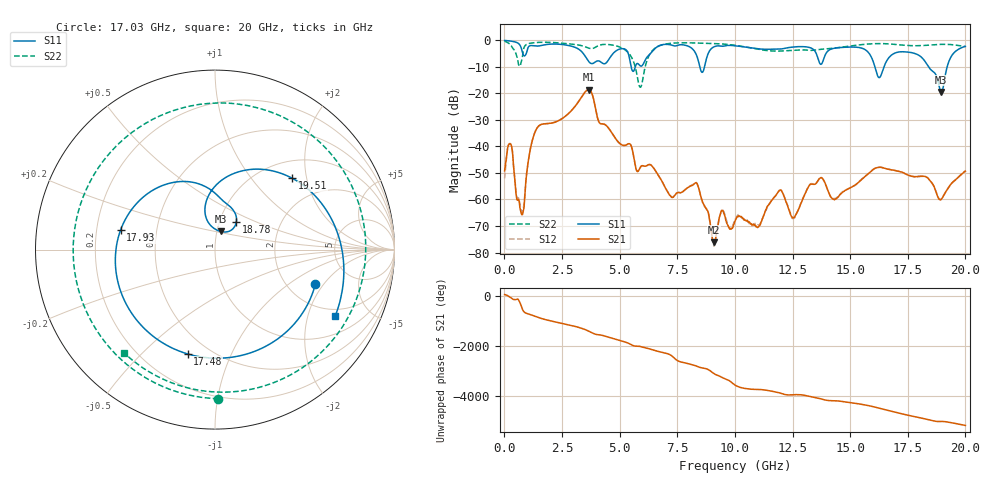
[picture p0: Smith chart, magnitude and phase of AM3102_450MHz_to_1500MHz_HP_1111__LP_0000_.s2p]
!Agilent Technologies,E8364B,MY43040894,A.07.50.67
!Agilent E8364B: A.07.50.67
!Date: Thursday, January 11, 2018 06:48:17
!Correction: S11(Full 2 Port(1,2))
!S21(Full 2 Port(1,2))
!S12(Full 2 Port(1,2))
!S22(Full 2 Port(1,2))
!S2P File: Measurements: S11, S21, S12, S22:
# Hz S  dB  R 50
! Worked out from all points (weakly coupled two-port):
!   1601 points, 10 MHz to 20 GHz, reference 50 ohm
!   highest |S21| = -18.60 dB at 3.658 GHz (marker M1); lowest = -76.1 dB at 9.08 GHz (marker M2)
!   lowest |S11| = -19.5 dB at 18.95 GHz (marker M3), VSWR 1.24, Z = 52.1 + j10.6 ohm
!   |S11| at or under -10 dB: 8.477 GHz to 8.682 GHz (204.6 MHz wide, 2.38 % of centre); 16.07 GHz to 16.47 GHz (396 MHz wide, 2.43 % of centre); 18.4 GHz to 19.21 GHz (809.2 MHz wide, 4.3 % of centre)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
!   |S22| runs from -17.7 to -0.4 dB; largest |S21 - S12| = 0.0015
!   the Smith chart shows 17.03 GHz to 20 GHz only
!   S11 on the Smith chart (normalised r, x): 17.03 GHz: 2.83, -1.65; 17.48 GHz: 0.38, -0.70; 17.93 GHz: 0.30, +0.09; 18.78 GHz: 1.20, +0.38; 19.51 GHz: 1.36, +1.65; 20 GHz: 1.68, -3.01
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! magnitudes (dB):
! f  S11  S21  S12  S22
! 10 MHz  -0.1  -49.3  -52.0  -0.4
! 259.9 MHz  -0.3  -39.1  -39.0  -1.6
! 772.1 MHz  -4.1  -65.8  -64.8  -6.6
! 1.384 GHz  -2.2  -33.6  -33.6  -0.8
! 3.346 GHz  -4.2  -21.4  -21.4  -2.0
! 3.658 GHz  -8.0  -18.6  -18.6  -2.9
! 5.895 GHz  -9.6  -47.9  -47.9  -17.7
! 6.682 GHz  -2.2  -50.9  -51.0  -2.2
! 8.343 GHz  -5.8  -53.9  -53.8  -1.0
! 9.08 GHz  -2.5  -76.1  -76.9  -1.2
! 10.01 GHz  -2.1  -68.2  -67.8  -1.9
! 11.97 GHz  -3.3  -56.4  -56.5  -4.1
! 12.55 GHz  -2.5  -66.8  -67.1  -3.8
! 13.34 GHz  -3.1  -54.2  -54.0  -3.8
! 16.68 GHz  -6.6  -48.6  -48.7  -1.4
! 17.03 GHz  -4.6  -49.2  -49.2  -1.6
! 17.48 GHz  -4.4  -50.7  -50.6  -1.9
! 17.93 GHz  -5.4  -51.4  -51.4  -2.0
! 18.78 GHz  -14.3  -58.4  -58.2  -1.6
! 18.95 GHz  -19.5  -60.0  -59.9  -1.5
! 19.51 GHz  -4.6  -53.0  -53.1  -1.7
! 20 GHz  -2.3  -49.3  -49.2  -2.3
